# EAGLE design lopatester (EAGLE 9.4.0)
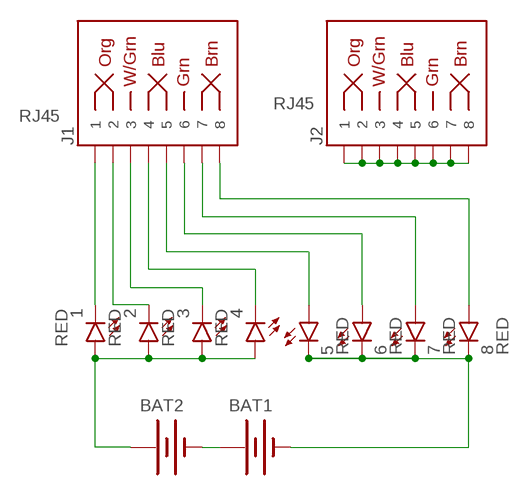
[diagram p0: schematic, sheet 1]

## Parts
1  RED  LED-RED1206  [LED-1206]
2  RED  LED-RED1206  [LED-1206]
3  RED  LED-RED1206  [LED-1206]
4  RED  LED-RED1206  [LED-1206]
5  RED  LED-RED1206  [LED-1206]
6  RED  LED-RED1206  [LED-1206]
7  RED  LED-RED1206  [LED-1206]
8  RED  LED-RED1206  [LED-1206]
BAT1  BATTERY20PTH  [BATTCOM_20MM_PTH]
BAT2  BATTERY20PTH  [BATTCOM_20MM_PTH]
J1  RJ45  RJ45-8  [RJ45-8]
J2  RJ45  RJ45-8  [RJ45-8]

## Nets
A1: 1.C J1.1
A2: 2.C J1.2
A3: 3.C J1.3
A4: 4.C J1.4
A5: 5.A J1.5
A6: 6.A J1.6
A7: 7.A J1.7
A8: 8.A J1.8
N$1: J2.1 J2.2 J2.3 J2.4 J2.5 J2.6 J2.7 J2.8
N$2: BAT1.1(+) BAT2.2(-)
N$3: 1.A 2.A 3.A 4.A BAT2.1(+)
N$4: 5.C 6.C 7.C 8.C BAT1.2(-)

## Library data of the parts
1-8 = SparkFun-LED:LED-RED: Assorted Red LEDs; PROD_ID: DIO-09912
BAT1 BAT2 = SparkFun-Electromechanical:BATTERY: Battery Holders
J1 J2 = SparkFun-Connectors:RJ45-8: RJ45 Jack - 8 pin Simple RJ45, 8-pin connection. Commonly used for Cat5, Cat5e, and Cat6 Ethernet cables. Here is the connector we sell at SparkFun: RJ45 8-Pin Connector (PRT-00643) Datasheet It is used on this SparkFun product: SparkFun RJ45 Breakout (BOB-00716) Note, you may also be interested in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; PROD_ID: CONN-08506; SF_ID: PRT-00643

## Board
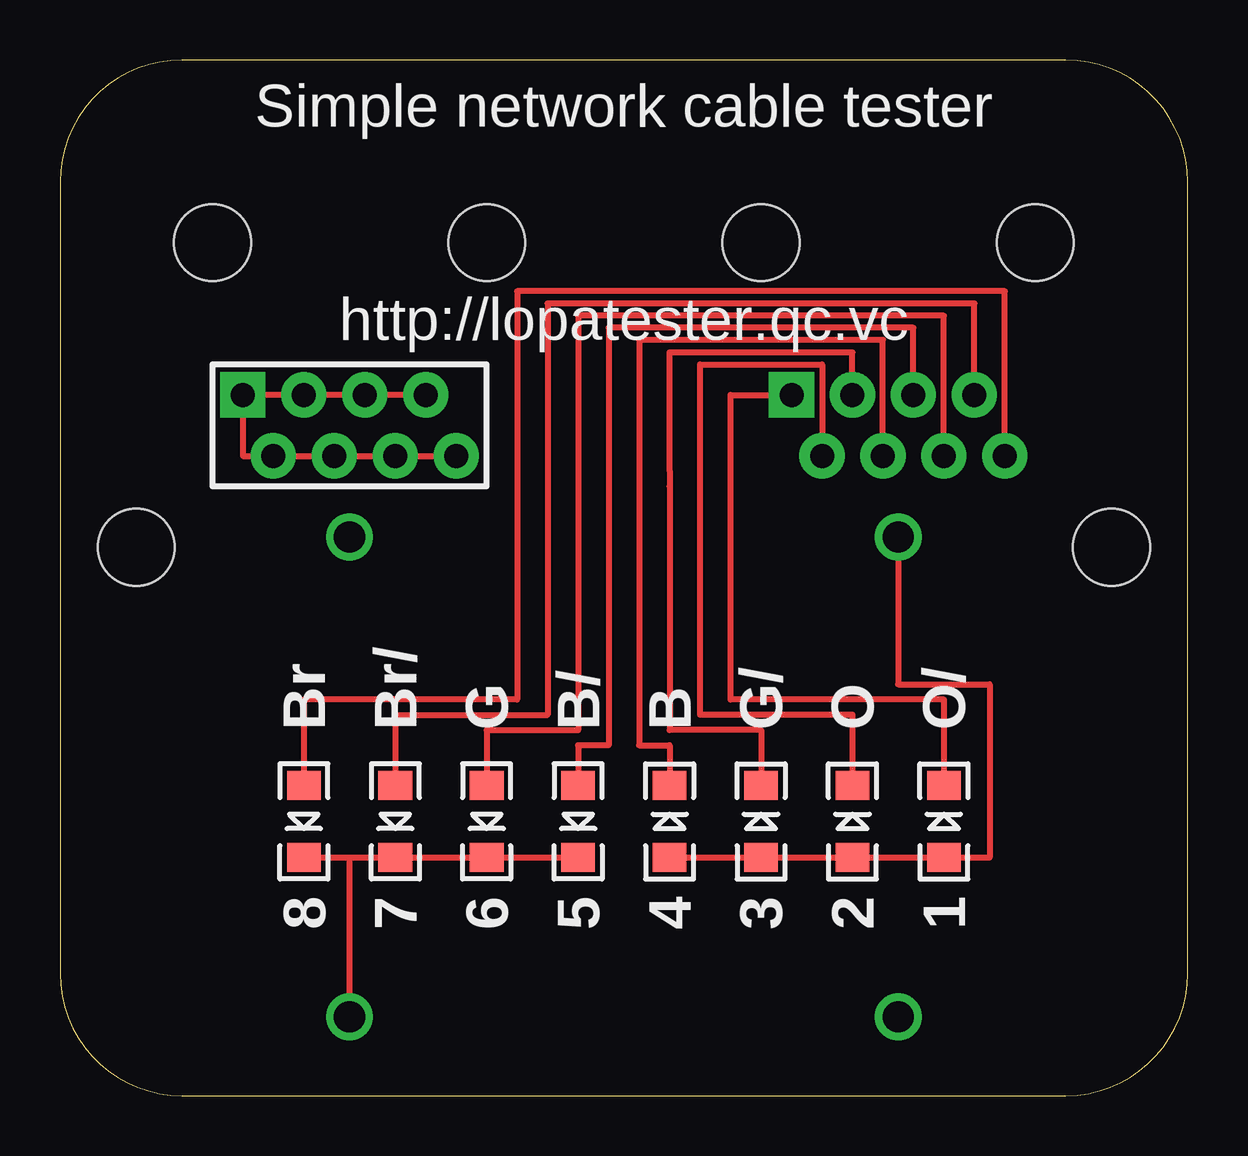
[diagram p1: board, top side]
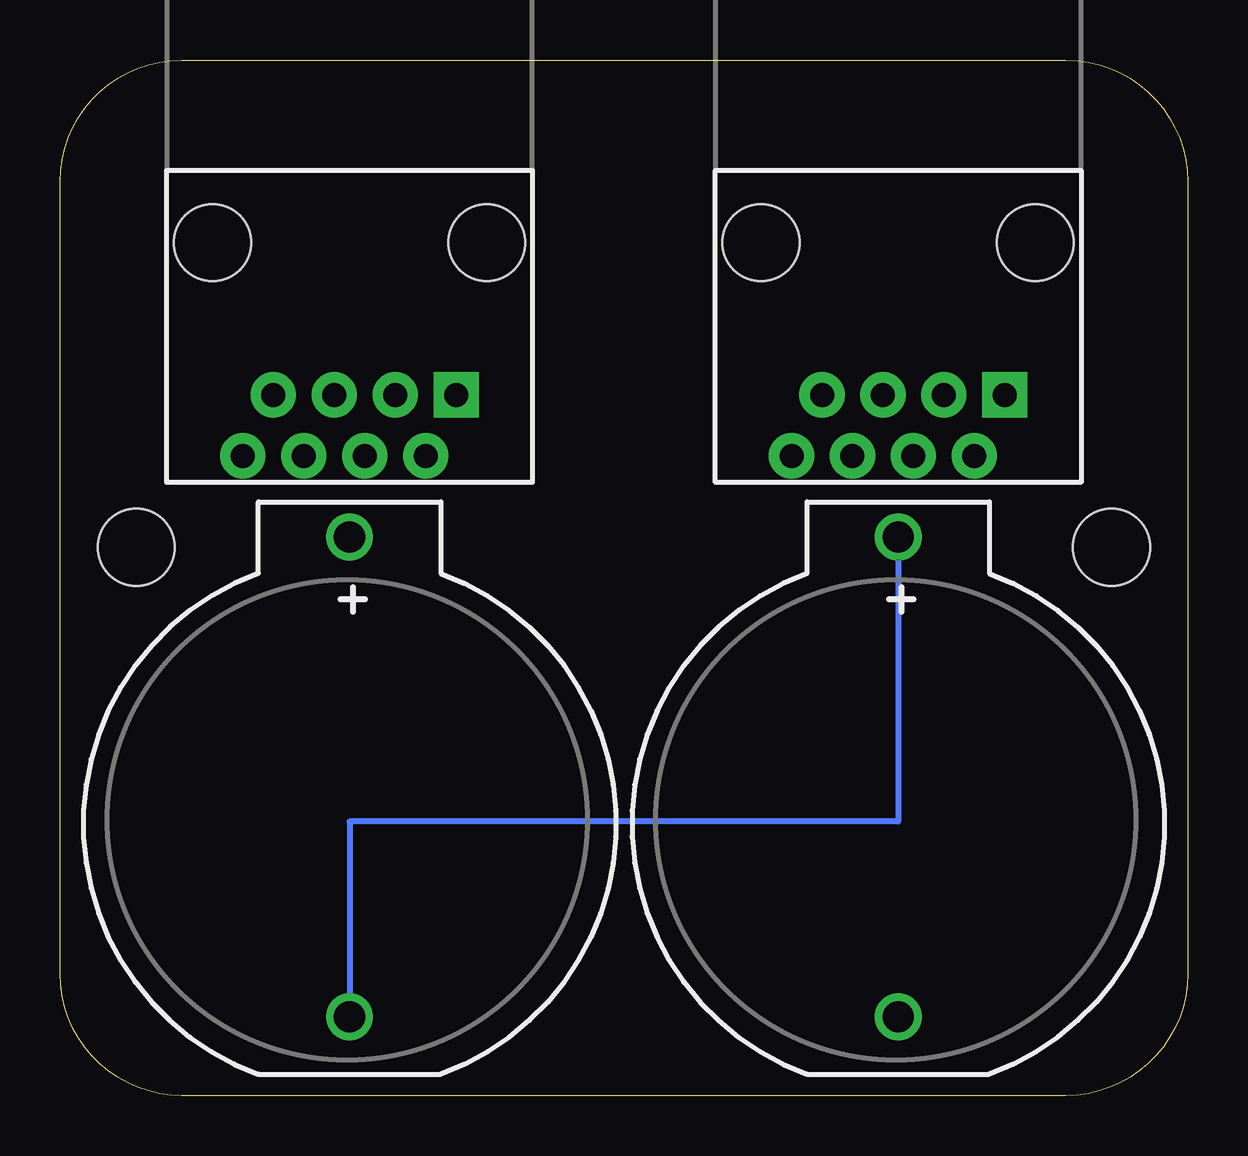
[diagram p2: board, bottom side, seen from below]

Size 46.99 x 43.17 mm. Coordinates in mm from the lower left corner, seen from the top.
Outline: 0,38.09 0,5.08 arc90 5.08,0 41.91,0 arc90 46.99,5.08 46.99,38.09 arc90 41.91,43.17 5.08,43.17 arc90 0,38.09
Copper layers (1*16): Top 0.035mm / dielectric 1.5mm / Bottom 0.035mm
Design rules "dirt_cheap_dirty_boards.v1": minimum track width 5mil, minimum drill 12mil, track to track 5mil, track to pad 5mil, pad to pad 5mil, via to via 5mil, smd to smd 0mil, copper to edge 10mil, drill to drill 10mil, minimum pad ring 10mil, minimum via ring 6mil, stop-mask expansion 2mil, vias tented up to drill 25mil, thermal gap 10mil
Holes 3.2 mm at 3.17,22.86 43.81,22.86

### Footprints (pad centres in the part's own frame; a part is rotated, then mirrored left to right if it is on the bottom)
LED-1206 = smd 1.2 x 1.4: A -1.5,0; C 1.5,0
BATTCOM_20MM_PTH = drill 1.3: 1 11.85,0; 2 -8.15,0
RJ45-8 = drill 1 pad 1.88 square: 1 -4.445,6.35 | drill 1 pad 1.88: 2 -3.175,8.89; 3 -1.905,6.35; 4 -0.635,8.89; 5 0.635,6.35; 6 1.905,8.89; 7 3.175,6.35; 8 4.445,8.89 | hole 3.2: -5.715,0; 5.715,0

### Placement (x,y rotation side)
1  36.83,11.43 90 top
2  33.02,11.43 90 top
3  29.21,11.43 90 top
4  25.4,11.43 90 top
5  21.59,11.43 270 top
6  17.78,11.43 270 top
7  13.97,11.43 270 top
8  10.16,11.43 270 top
BAT1  12.06,11.43 90 bottom
BAT2  34.92,11.43 90 bottom
J1  34.92,35.56 180 bottom
J2  12.06,35.56 180 bottom

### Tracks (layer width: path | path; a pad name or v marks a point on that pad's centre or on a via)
A1
  Top 0.254: 1.C 36.83,16.51 27.94,16.51 27.94,29.21 J1.1
A2
  Top 0.254: 2.C 33.02,15.88 26.67,15.88 26.67,30.48 31.75,30.48 J1.2
A3
  Top 0.254: 3.C 29.21,15.24 25.4,15.24 25.4,25.4 25.4,26.04 25.4,30.99 33.02,30.99 J1.3
A4
  Top 0.254: 4.C 25.4,14.61 24.13,14.61 24.13,31.5 34.29,31.5 J1.4
A5
  Top 0.254: 5.A 21.59,14.61 22.86,14.61 22.86,32 35.56,32 J1.5
A6
  Top 0.254: J1.6 36.83,32.51 21.59,32.51 21.59,15.24 17.78,15.24 6.A 17.78,12.7
A7
  Top 0.254: 7.A 13.97,15.88 20.32,15.88 20.32,33.02 38.1,33.02 J1.7
A8
  Top 0.254: J1.8 39.37,33.53 19.05,33.53 19.05,16.51 10.16,16.51 8.A
N$1
  Top 0.254: J2.7 J2.5 J2.3 J2.1 7.62,26.67 J2.2 J2.4 J2.6 J2.8
N$2
  Bottom 0.254: BAT1.1 12.06,11.43 34.92,11.43 BAT2.2
N$3
  Top 0.254: 4.A 3.A 2.A 1.A 38.73,9.93 38.73,17.14 34.92,17.14 BAT2.1
N$4
  Top 0.254: BAT1.2 12.06,9.93 | 8.C 12.06,9.93 | 12.06,9.93 7.C 6.C 5.C

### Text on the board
tPlace: Simple network cable tester | http://lopatester.qc.vc | Br | Br/ | G | B/ | B | G/ | O | O/

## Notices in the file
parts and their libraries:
SparkFun-Electromechanical: Licensing: Creative Commons ShareAlike 4.0 International - https://creativecommons.org/licenses/by-sa/4.0
